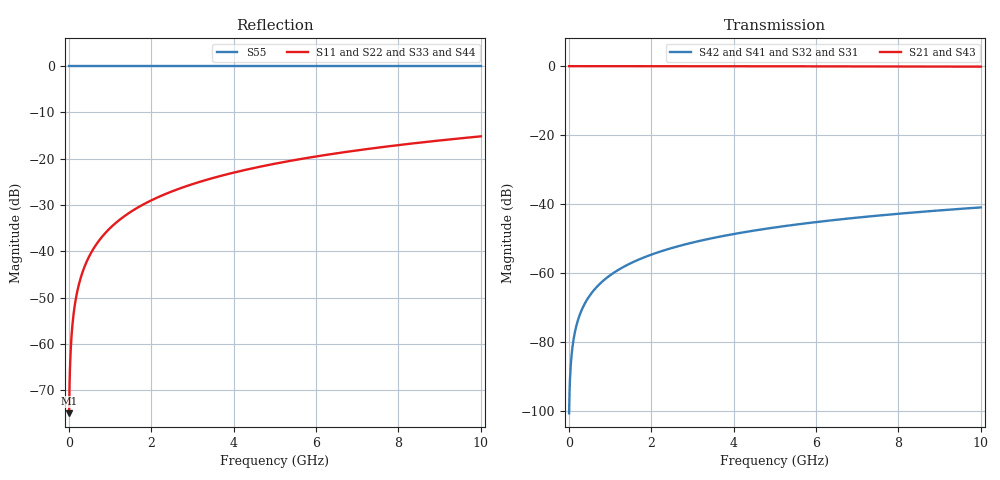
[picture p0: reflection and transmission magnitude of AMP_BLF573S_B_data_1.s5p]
! Created Thu Sep 17 17:28:06 2009
# hz S ma R 50
! 5 Port Network Data from SP1.SP block
! freq  magS11  angS11  magS12  angS12  magS13  angS13  magS14  angS14
!  magS15  angS15
!  magS21  angS21  magS22  angS22  magS23  angS23
!  magS24  angS24  magS25  angS25
!  magS31  angS31  magS32  angS32
!  magS33  angS33  magS34  angS34  magS35  angS35
!  magS41  angS41
!  magS42  angS42  magS43  angS43  magS44  angS44  magS45  angS45
!  magS51  angS51  magS52  angS52  magS53  angS53  magS54  angS54
!  magS55  angS55
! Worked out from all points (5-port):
!   1000 points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, 10 MHz to 10 GHz, reference 50 ohm
!   strongest paths, dB at 10 MHz, 2.51 GHz, 5.01 GHz, 7.51 GHz, 10 GHz:
!     S21: 0.0, 0.0, 0.0, -0.1, -0.1
!     S43: 0.0, 0.0, 0.0, -0.1, -0.1
!     S42: -100.7, -52.7, -46.8, -43.3, -41.0
!     S41: -100.7, -52.7, -46.8, -43.3, -41.0
!     S32: -100.7, -52.7, -46.8, -43.3, -41.0
!     S31: -100.7, -52.7, -46.8, -43.3, -41.0
!   lowest |S11| = -75.0 dB at 10 MHz (marker M1), VSWR 1.00, Z = 50 + j0.0177 ohm
!   |S11| at or under -10 dB: start of sweep to end of sweep
